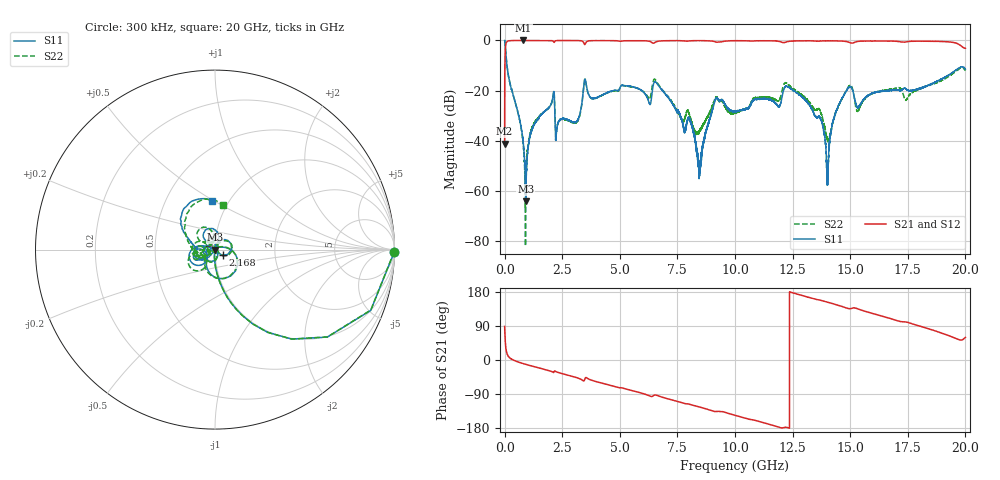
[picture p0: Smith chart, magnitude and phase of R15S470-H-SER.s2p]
!{R15S470}
!Johanson Technology Inc.
!www.johansontechnology.com
!Test Board Conditions:
!Substrate Type  RO4350B
!Substrate Thickness  20 mil
!Substrate Dk  3.66
!TL Type: GCPW
!TL Trace Width  34 mil
!TL Gap  10 mil
!Electrode orientation  Horizontal
!DUT TOPOLOGY	SERIES
!Mounting Pad LxW  26x52 mil
! Created Sat Feb  6 14:30:21 2021
# hz S ma R 50
! 2 Port Network Data from SP1.SP block
! freq  magS11  angS11  magS21  angS21  magS12  angS12  magS22  angS22
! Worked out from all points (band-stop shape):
!   20001 points, 300 kHz to 20 GHz, reference 50 ohm
!   highest |S21| = 0.00 dB at 816.3 MHz (marker M1); lowest = -41.2 dB at 300 kHz (marker M2)
!   |S21| within 3 dB of the highest: 34.51 MHz to 19.94 GHz (19.91 GHz wide, 199 % of centre)
!   lowest |S11| = -64.1 dB at 915.3 MHz (marker M3), VSWR 1.00, Z = 49.9 + j0.0102 ohm
!   |S11| at or under -10 dB: 101.8 MHz to end of sweep
!   |S22| runs from -82.0 to 0.0 dB; largest |S21 - S12| = 0.014
!   S11 on the Smith chart (normalised r, x): 300 kHz: open; 2.168 GHz: 1.09, -0.07; 20 GHz: 0.85, +0.48
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300000  0.999 -0.8  0.008727 88.7  0.008741 89.3  0.9984 -0.7
1.213e8  0.2683 -75.8  0.962 14.0  0.9624 13.9  0.2692 -75.9
8.163e8  0.008486 -102.5  0.9999 -9.6  0.9984 -9.6  0.007893 -99.0
9.153e8  0.0006269 170.6  0.9996 -11.4  0.9993 -11.4  0.0009183 65.3
1.2693e9  0.0205 78.0  0.999 -17.3  0.999 -17.3  0.02175 70.0
2.1683e9  0.05599 -34.8  0.9397 -28.7  0.9402 -28.7  0.06145 -36.4
3.3343e9  0.04892 16.1  0.9807 -51.6  0.9805 -51.6  0.04692 20.2
3.5073e9  0.1644 -80.3  0.8591 -46.9  0.8598 -46.8  0.1622 -84.3
6.6673e9  0.1285 179.5  0.9664 -94.6  0.9666 -94.5  0.1339 -168.7
8.0503e9  0.02566 164.1  0.982 -117.1  0.9827 -117.1  0.02968 -159.4
8.4493e9  0.002377 64.8  0.9906 -123.9  0.9909 -123.8  0.0156 -96.5
9.1693e9  0.06919 -108.1  0.928 -136.0  0.9305 -136.1  0.07438 -111.7
1.00003e10  0.03871 138.8  0.9883 -146.0  0.9883 -146.0  0.03573 124.8
1.22063e10  0.1222 112.2  0.9273 -177.6  0.9242 -177.7  0.1429 122.1
1.33343e10  0.04247 67.5  0.9821 163.1  0.9825 163.0  0.04902 95.7
1.37423e10  0.02627 80.0  0.9752 157.3  0.9762 157.3  0.0344 98.8
1.40123e10  0.002571 146.8  0.9829 152.6  0.9817 152.7  0.01058 137.4
1.43163e10  0.03051 -128.2  0.98 147.2  0.9821 147.1  0.02947 -141.8
1.49153e10  0.1121 -152.5  0.9296 135.9  0.9276 135.8  0.1175 -163.1
1.53323e10  0.04538 -167.5  0.9559 134.9  0.9542 135.0  0.03846 -173.9
1.66673e10  0.09929 -154.9  0.9764 110.6  0.9662 110.7  0.1049 -161.0
2e10  0.2661 92.9  0.7019 59.6  0.6982 59.6  0.2492 79.1
